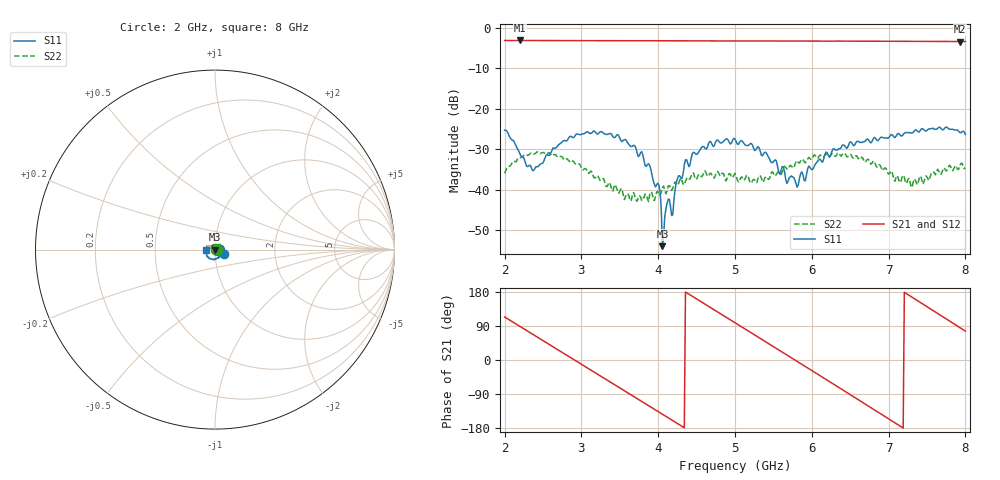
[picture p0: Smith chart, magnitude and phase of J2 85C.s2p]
!Agilent Technologies,E8364B,MY43040699,A.07.50.67
!Agilent E8364B: A.07.50.67
!Date: Friday, June 06, 2025 09:28:39
!Correction: S11(Full 2 Port(1,2))
!S21(Full 2 Port(1,2))
!S12(Full 2 Port(1,2))
!S22(Full 2 Port(1,2))
!S2P File: Measurements: S11, S21, S12, S22:
# Hz S  dB  R 50
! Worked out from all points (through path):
!   401 points, 2 GHz to 8 GHz, reference 50 ohm
!   highest |S21| = -3.19 dB at 2.195 GHz (marker M1); lowest = -3.5 dB at 7.925 GHz (marker M2)
!   group delay of S21, straight-line fit = 350 ps
!   lowest |S11| = -53.9 dB at 4.055 GHz (marker M3), VSWR 1.00, Z = 49.8 - j0.0951 ohm
!   |S11| at or under -10 dB: start of sweep to end of sweep
!   |S22| runs from -43.0 to -30.7 dB; largest |S21 - S12| = 0.0072
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2e9  -25.32 -28.1  -3.19 113.6  -3.20 113.7  -35.93 -12.9
2.195e9  -30.91 -30.3  -3.19 89.2  -3.21 89.3  -32.09 -36.5
2.39e9  -34.96 11.7  -3.20 64.9  -3.21 65.0  -31.20 -60.0
2.72e9  -28.67 33.3  -3.22 23.7  -3.25 23.7  -31.82 -105.5
3.005e9  -26.25 14.9  -3.23 -11.8  -3.27 -11.8  -34.84 -149.2
3.53e9  -28.13 -34.2  -3.25 -77.3  -3.31 -77.1  -40.06 135.0
3.785e9  -30.62 -63.2  -3.26 -109.2  -3.31 -109.0  -42.66 105.0
4.01e9  -38.98 -109.1  -3.26 -137.4  -3.31 -137.1  -41.33 93.9
4.055e9  -53.93 -151.7  -3.26 -143.0  -3.32 -142.6  -39.53 103.1
4.19e9  -46.14 107.8  -3.27 -159.9  -3.32 -159.5  -39.68 92.2
4.25e9  -37.26 88.4  -3.28 -167.5  -3.31 -167.0  -38.90 80.7
4.46e9  -30.76 50.0  -3.28 166.2  -3.32 166.7  -35.86 59.1
5e9  -27.47 -26.7  -3.31 98.4  -3.32 98.9  -35.98 -22.8
5.27e9  -30.22 -59.8  -3.32 64.5  -3.32 64.9  -38.17 -95.2
5.555e9  -34.28 -129.9  -3.32 28.4  -3.32 28.9  -35.64 -149.5
5.81e9  -39.39 149.1  -3.33 -3.8  -3.32 -3.4  -32.95 157.6
6.005e9  -35.04 83.4  -3.34 -28.5  -3.33 -28.1  -32.33 135.7
6.5e9  -28.19 3.6  -3.35 -91.4  -3.35 -91.0  -31.27 82.7
7.01e9  -27.01 -50.0  -3.39 -156.5  -3.37 -156.2  -36.14 62.9
7.415e9  -25.35 -91.4  -3.41 151.6  -3.39 151.9  -36.62 78.9
7.925e9  -25.87 -161.0  -3.45 85.8  -3.41 86.1  -34.29 66.6
8e9  -26.35 -174.0  -3.45 76.1  -3.41 76.3  -34.64 61.6
